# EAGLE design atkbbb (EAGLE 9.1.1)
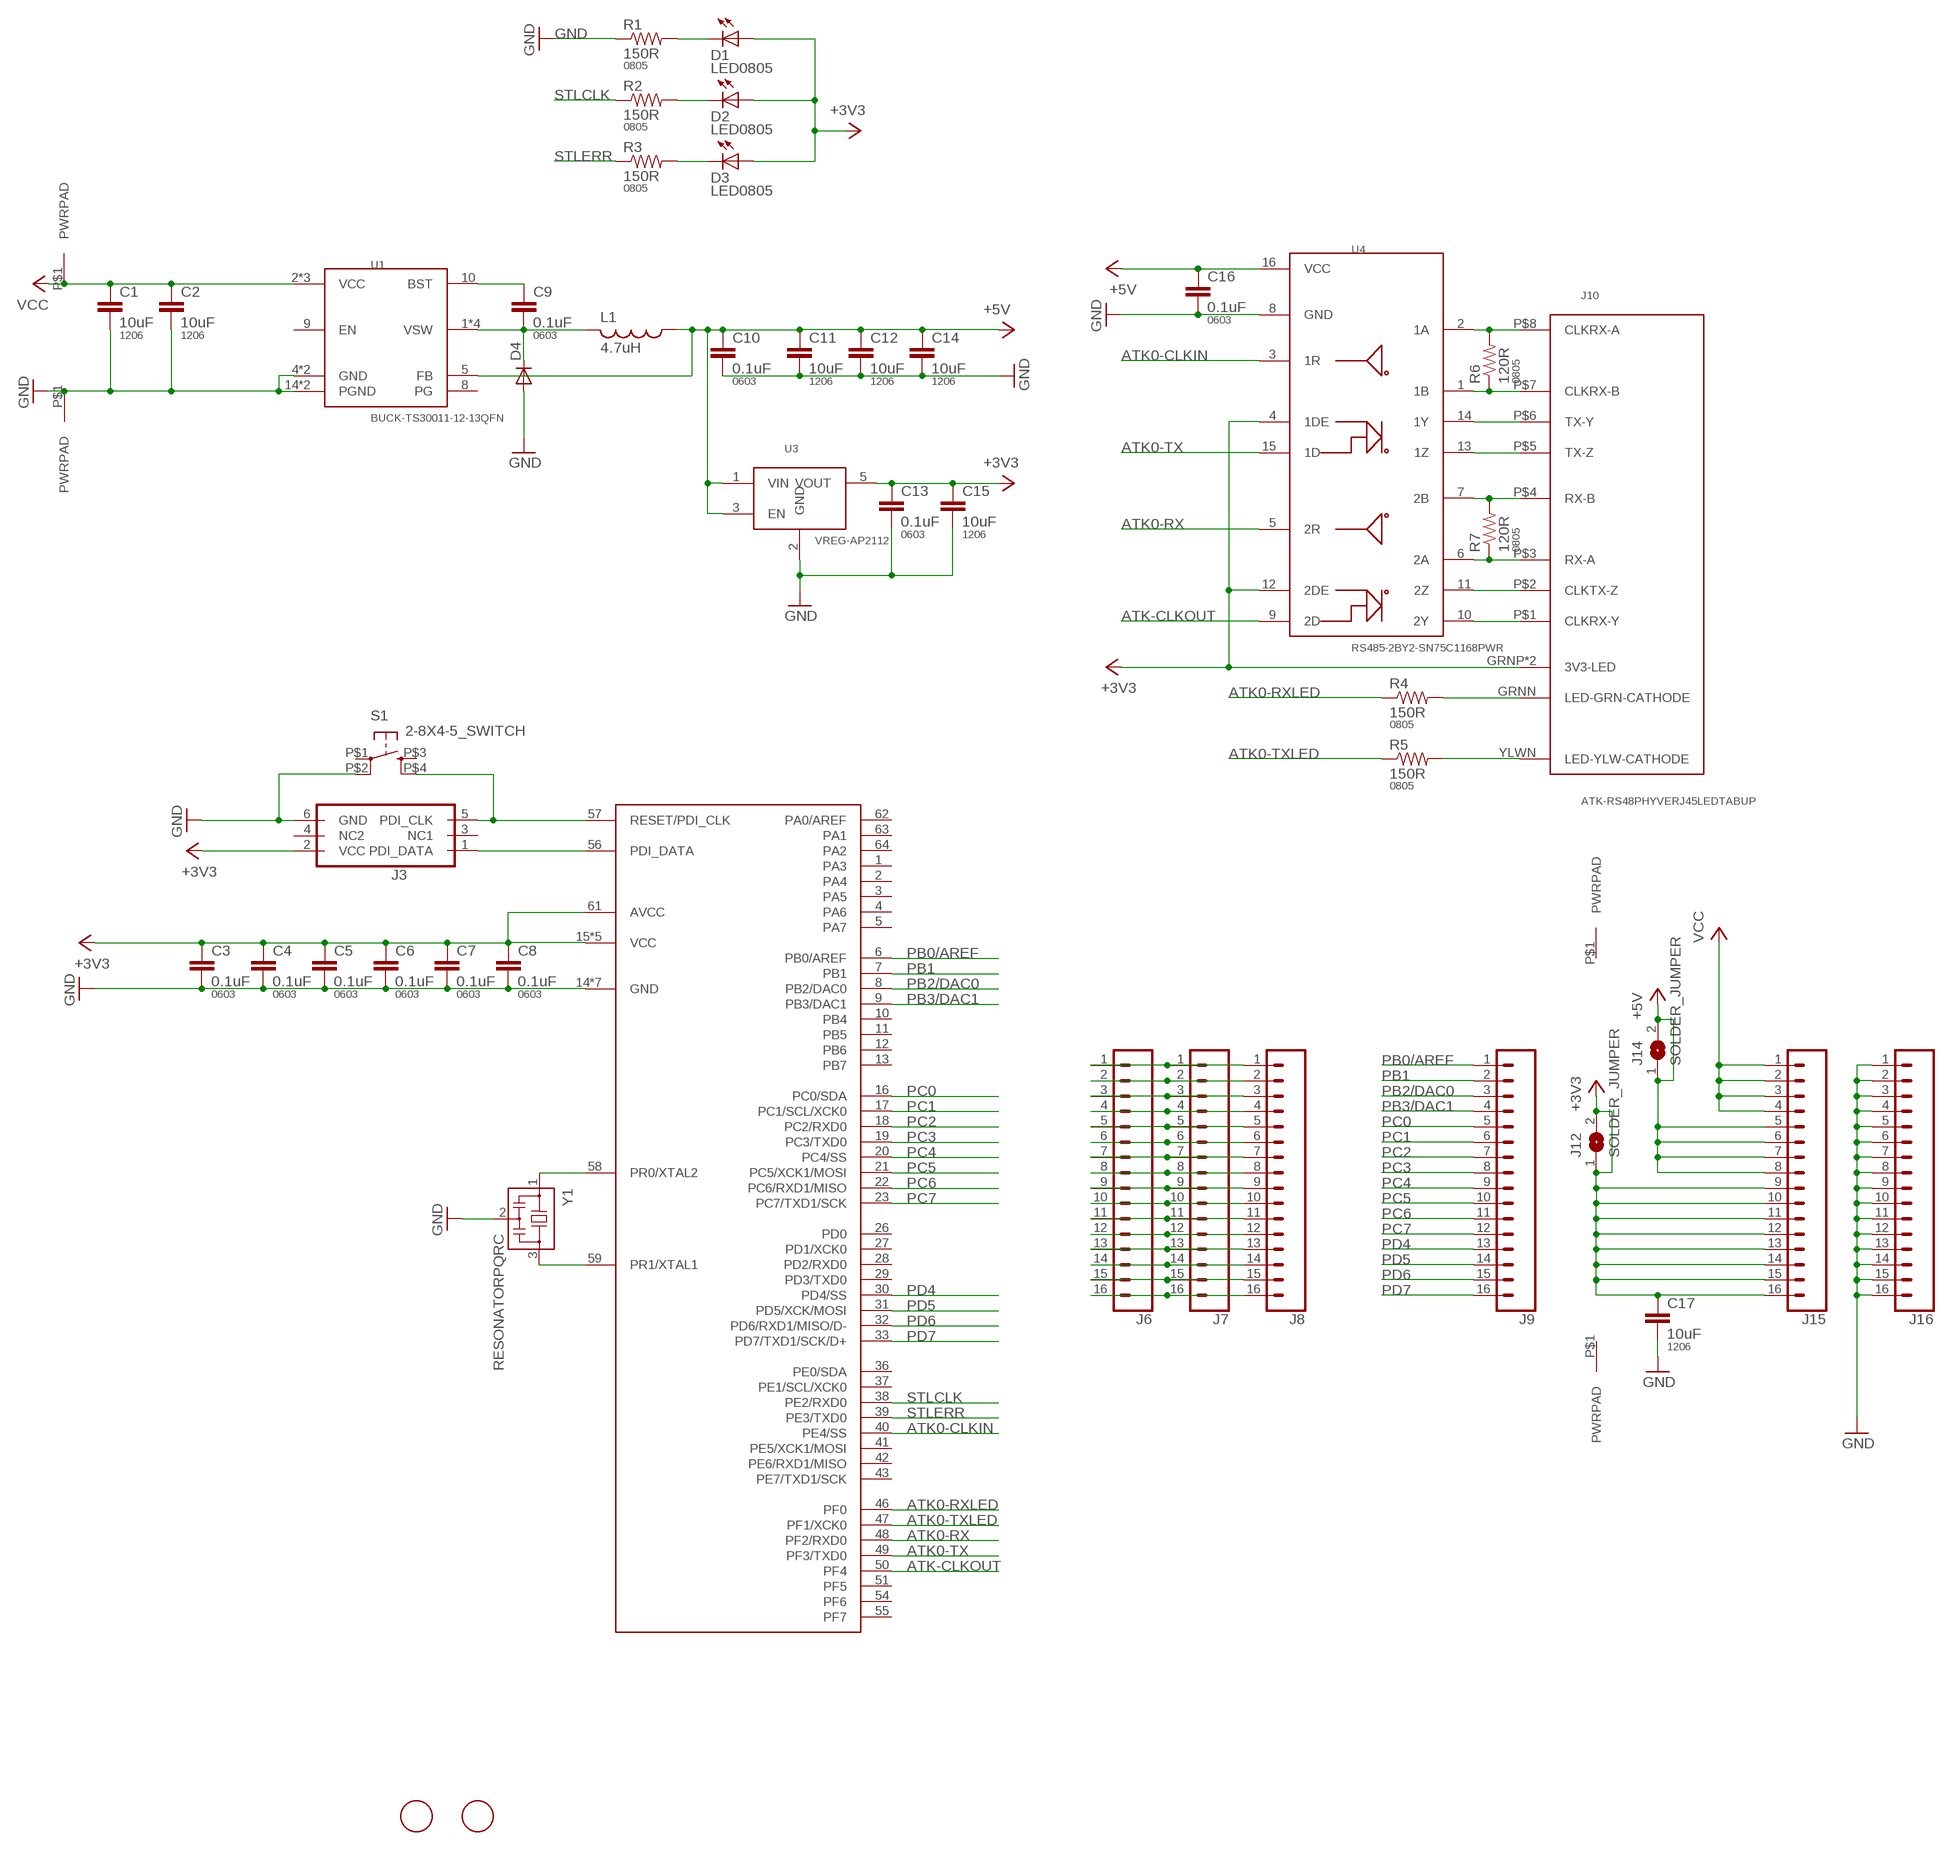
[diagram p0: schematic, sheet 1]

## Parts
C1  10uF  CAP1206  [1206]
C2  10uF  CAP1206  [1206]
C3  0.1uF  CAP0603-CAP  [0603-CAP]
C4  0.1uF  CAP0603-CAP  [0603-CAP]
C5  0.1uF  CAP0603-CAP  [0603-CAP]
C6  0.1uF  CAP0603-CAP  [0603-CAP]
C7  0.1uF  CAP0603-CAP  [0603-CAP]
C8  0.1uF  CAP0603-CAP  [0603-CAP]
C9  0.1uF  CAP0603-CAP  [0603-CAP]
C10  0.1uF  CAP0603-CAP  [0603-CAP]
C11  10uF  CAP1206  [1206]
C12  10uF  CAP1206  [1206]
C13  0.1uF  CAP0603-CAP  [0603-CAP]
C14  10uF  CAP1206  [1206]
C15  10uF  CAP1206  [1206]
C16  0.1uF  CAP0603-CAP  [0603-CAP]
C17  10uF  CAP1206  [1206]
D1  LED0805  [LED0805]
D2  LED0805  [LED0805]
D3  LED0805  [LED0805]
D4  DIODESOD123HE  [SOD-123HE]
J1  PWRPADM3-STANDOFF  [PWRPAD_M3_STANDOFF]
J2  PWRPADM3-STANDOFF  [PWRPAD_M3_STANDOFF]
J3  PDIFEMALE_SMD  [PDI_2X3_SMD]
J4  FIDUCIAL  [FIDUCIAL_1MM]
J5  FIDUCIAL  [FIDUCIAL_1MM]
J6  CONN_161X16_NO_SILK  [1X16_NO_SILK]
J7  CONN_161X16_NO_SILK  [1X16_NO_SILK]
J8  CONN_161X16_NO_SILK  [1X16_NO_SILK]
J9  CONN_161X16_NO_SILK  [1X16_NO_SILK]
J10  ATK-RS48PHYVERJ45LEDTABUP  [RJ45-LED-RJHSE-5381-UPTAB]
J11  PWRPADM3  [PWRPAD_3-25MM]
J12  SOLDER_JUMPER  [SJFAB]
J13  PWRPADM3  [PWRPAD_3-25MM]
J14  SOLDER_JUMPER  [SJFAB]
J15  CONN_161X16_NO_SILK  [1X16_NO_SILK]
J16  CONN_161X16_NO_SILK  [1X16_NO_SILK]
L1  4.7uH  INDUCTOR  [NRS5020T4R7MMGJ]
R1  150R  RESISTOR0805-RES  [0805]
R2  150R  RESISTOR0805-RES  [0805]
R3  150R  RESISTOR0805-RES  [0805]
R4  150R  RESISTOR0805-RES  [0805]
R5  150R  RESISTOR0805-RES  [0805]
R6  120R  RESISTOR0805-RES  [0805]
R7  120R  RESISTOR0805-RES  [0805]
S1  2-8X4-5_SWITCH  [TACT-SWITCH-KMR6]
U1  BUCK-TS30011-12-13QFN  [QFN16-3X3-TI-RTE]
U2  ATXMEGA_A3UQFN  [QFN-64-9X9MM]
U3  VREG-AP2112  [SOT23-5]
U4  RS485-2BY2-SN75C1168PWR  [TSSOP16]
Y1  RESONATORPQRC  [RES_PRQC]

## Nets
+3V3: C3.1 C4.1 C5.1 C6.1 C7.1 C8.1 C13.1 C15.1 C17.1 D1.1(A) D2.1(A) D3.1(A) J3.2(VCC) J10.GRNP(3V3-LED) J10.YLWP(3V3-LED) J12.1 J12.2 J15.9 J15.10 J15.11 J15.12 J15.13 J15.14 J15.15 J15.16 U2.15(VCC) U2.25(VCC) U2.35(VCC) U2.45(VCC) U2.53(VCC) U2.61(AVCC) U3.5(VOUT) U4.4(1DE) U4.12(2DE)
+5V: C10.1 C11.1 C12.1 C14.1 C16.1 J14.1 J14.2 J15.5 J15.6 J15.7 J15.8 L1.1 U1.5(FB) U3.1(VIN) U3.3(EN) U4.16(VCC)
ATK0-CLKIN: U2.40(PE4/SS) U4.3(1R)
ATK0-RX: U2.48(PF2/RXD0) U4.5(2R)
ATK0-RXLED: R4.1 U2.46(PF0)
ATK0-TX: U2.49(PF3/TXD0) U4.15(1D)
ATK0-TXLED: R5.1 U2.47(PF1/XCK0)
ATK-CLKOUT: U2.50(PF4) U4.9(2D)
GND: C1.2 C2.2 C3.2 C4.2 C5.2 C6.2 C7.2 C8.2 C10.2 C11.2 C12.2 C13.2 C14.2 C15.2 C16.2 C17.2 D4.P$2(A) J2.P$1(PWRPAD) J3.6(GND) J16.1 J16.2 J16.3 J16.4 J16.5 J16.6 J16.7 J16.8 J16.9 J16.10 J16.11 J16.12 J16.13 J16.14 J16.15 J16.16 R1.1 S1.P$2(P1) U1.4(GND) U1.14(PGND) U1.15(PGND) U1.TH(GND) U2.14(GND) U2.24(GND) U2.34(GND) U2.44(GND) U2.52(GND) U2.60(GND) U2.P$1(GND) U3.2(GND) U4.8(GND) Y1.2
N$1: U2.58(PR0/XTAL2) Y1.1
N$2: U2.59(PR1/XTAL1) Y1.3
N$3: J3.5(PDI_CLK) S1.P$4(S1) U2.57(RESET/PDI_CLK)
N$4: J3.1(PDI_DATA) U2.56(PDI_DATA)
N$5: C9.1 U1.10(BST)
N$6: C9.2 D4.P$1(C) L1.2 U1.1(VSW) U1.12(VSW) U1.13(VSW) U1.16(VSW)
N$7: J10.GRNN(LED-GRN-CATHODE) R4.2
N$8: J10.P$8(CLKRX-A) R6.2 U4.2(1A)
N$9: D1.2(C) R1.2
N$10: D2.2(C) R2.2
N$11: D3.2(C) R3.2
N$12: J10.P$7(CLKRX-B) R6.1 U4.1(1B)
N$13: J10.P$6(TX-Y) U4.14(1Y)
N$14: J10.P$5(TX-Z) U4.13(1Z)
N$15: J10.P$4(RX-B) R7.2 U4.7(2B)
N$16: J10.P$3(RX-A) R7.1 U4.6(2A)
N$17: J10.P$2(CLKTX-Z) U4.11(2Z)
N$18: J10.P$1(CLKRX-Y) U4.10(2Y)
N$19: J10.YLWN(LED-YLW-CATHODE) R5.2
N$20: J6.1 J7.1 J8.1
N$21: J6.2 J7.2 J8.2
N$22: J6.3 J7.3 J8.3
N$23: J6.4 J7.4 J8.4
N$24: J6.5 J7.5 J8.5
N$25: J6.6 J7.6 J8.6
N$26: J6.7 J7.7 J8.7
N$27: J6.8 J7.8 J8.8
N$28: J6.9 J7.9 J8.9
N$29: J6.10 J7.10 J8.10
N$30: J6.11 J7.11 J8.11
N$31: J6.12 J7.12 J8.12
N$32: J6.13 J7.13 J8.13
N$33: J6.14 J7.14 J8.14
N$34: J6.15 J7.15 J8.15
N$35: J6.16 J7.16 J8.16
PB0/AREF: J9.1 U2.6(PB0/AREF)
PB1: J9.2 U2.7(PB1)
PB2/DAC0: J9.3 U2.8(PB2/DAC0)
PB3/DAC1: J9.4 U2.9(PB3/DAC1)
PC0: J9.5 U2.16(PC0/SDA)
PC1: J9.6 U2.17(PC1/SCL/XCK0)
PC2: J9.7 U2.18(PC2/RXD0)
PC3: J9.8 U2.19(PC3/TXD0)
PC4: J9.9 U2.20(PC4/SS)
PC5: J9.10 U2.21(PC5/XCK1/MOSI)
PC6: J9.11 U2.22(PC6/RXD1/MISO)
PC7: J9.12 U2.23(PC7/TXD1/SCK)
PD4: J9.13 U2.30(PD4/SS)
PD5: J9.14 U2.31(PD5/XCK/MOSI)
PD6: J9.15 U2.32(PD6/RXD1/MISO/D-)
PD7: J9.16 U2.33(PD7/TXD1/SCK/D+)
STLCLK: R2.1 U2.38(PE2/RXD0)
STLERR: R3.1 U2.39(PE3/TXD0)
VCC: C1.1 C2.1 J1.P$1(PWRPAD) J15.1 J15.2 J15.3 J15.4 U1.2(VCC) U1.3(VCC) U1.11(VCC)
Unconnected: J3.3(NC1) J3.4(NC2) J11.P$1(PWRPAD) J13.P$1(PWRPAD) S1.P$1(P) S1.P$3(S) U1.8(PG) U1.9(EN) U2.1(PA3) U2.2(PA4) U2.3(PA5) U2.4(PA6) U2.5(PA7) U2.10(PB4) U2.11(PB5) U2.12(PB6) U2.13(PB7) U2.26(PD0) U2.27(PD1/XCK0) U2.28(PD2/RXD0) U2.29(PD3/TXD0) U2.36(PE0/SDA) U2.37(PE1/SCL/XCK0) U2.41(PE5/XCK1/MOSI) U2.42(PE6/RXD1/MISO) U2.43(PE7/TXD1/SCK) U2.51(PF5) U2.54(PF6) U2.55(PF7) U2.62(PA0/AREF) U2.63(PA1) U2.64(PA2)

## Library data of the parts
C1 C2 C11 C12 C14 C15 C17 = borkedlabs-passives:CAP: Capacitor; PACKAGE: 1206
C3-C10 C13 C16 = borkedlabs-passives:CAP: Capacitor; PACKAGE: 0603
D1-D3 = lights:LED: LED
D4 = passives:DIODE: DIODE
J1 J2 J11 J13 = power:PWRPAD
J3 = microcontrollers:PDI: Multi connection point. Often used as Generic Header-pin footprint for 0.1 inch spaced/style header connections You can populate with any combo of single row headers, but if you'd like an exact match, check these: Header - 2x3 (Male, 0.1") (PRT-12807) Header - 2x3 (Female, 0.1") (PRT-13010) 2x3 Pin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; PROD_ID: CONN-11290
J4 J5 = connector:FIDUCIAL: For use by pick and place machines to calibrate the vision/machine, 1mm
J6-J9 J15 J16 = SparkFun-Connectors:CONN_16: Multi connection point. Often used as Generic Header-pin footprint for 0.1 inch spaced/style header connections On any of the 0.1 inch spaced packages, you can populate with these: Break Away Headers - Straight (PRT-00116) Break Away Male Headers - Right Angle (PRT-00553) Female Headers (PRT-00115)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
J10 = connector:ATK-RS48PHYVE
J12 J14 = connector:SOLDER_JUMPER
L1 = power:INDUCTOR
R1-R7 = borkedlabs-passives:RESISTOR: Resistor; PACKAGE: 0805
S1 = passives:2-8X4-5_SWITCH
U1 = power:BUCK-TS30011-12-13
U2 = microcontrollers:ATXMEGA_A3U
U3 = power:VREG-AP2112
U4 = comm:RS485-2BY2-SN75C1168PWR
Y1 = passives:RESONATOR

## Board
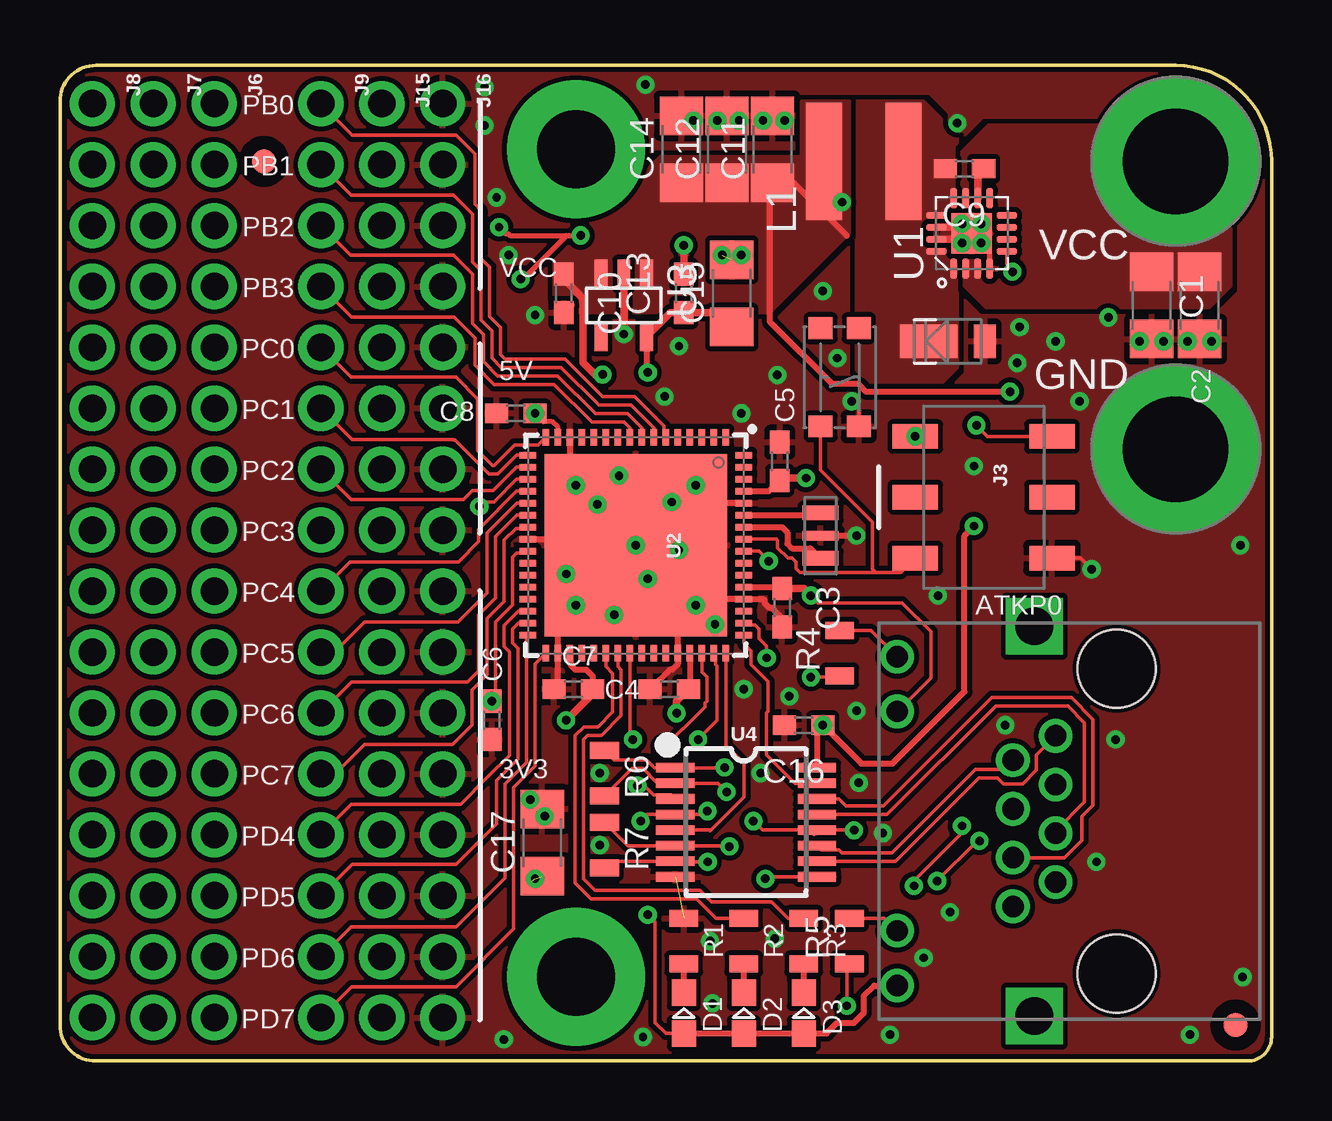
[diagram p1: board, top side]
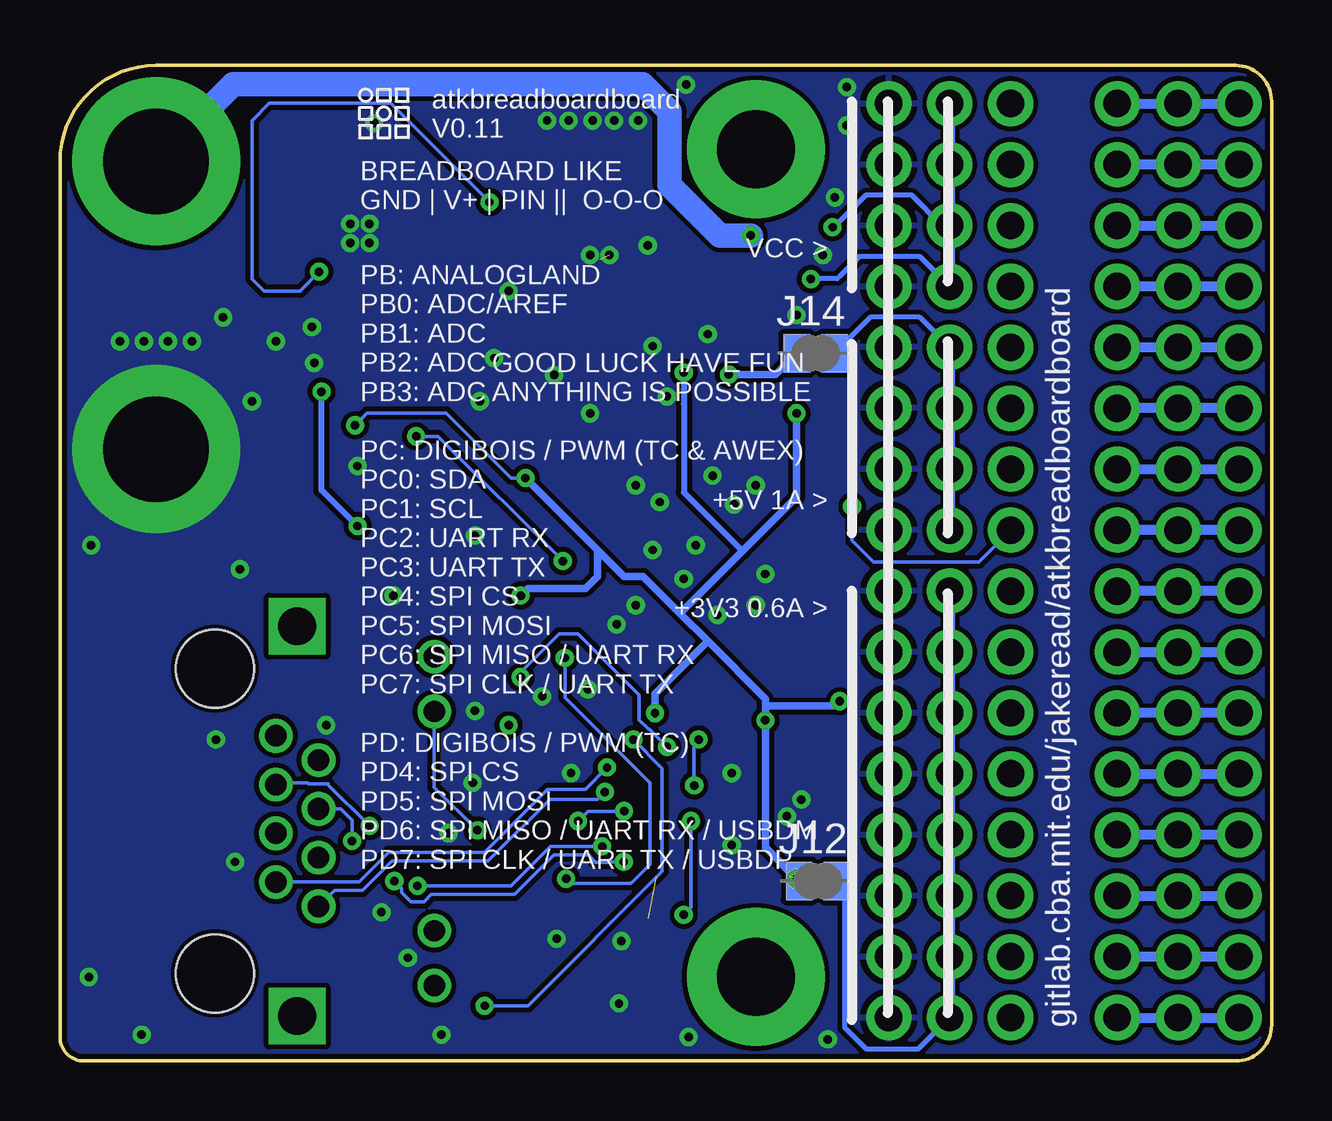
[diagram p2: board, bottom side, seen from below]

Size 50.5 x 41.5 mm. Coordinates in mm from the lower left corner, seen from the top.
Outline: 46.5,41.5 1.5,41.5 arc90 0,40 0,1.5 arc90 1.5,0 49.5,0 arc90 50.5,1 50.5,37.5 arc90 46.5,41.5
Copper layers (1*16): Top 0.035mm / dielectric 1.5mm / Bottom 0.035mm
Design rules "default *": minimum track width 6mil, minimum drill 0.35mm, track to track 8mil, track to pad 8mil, pad to pad 8mil, via to via 8mil, smd to smd 8mil, copper to edge 8mil, drill to drill 8mil, minimum pad ring 10mil, minimum via ring 8mil, stop-mask expansion 4mil, vias tented up to drill 25mil, thermal gap 10mil

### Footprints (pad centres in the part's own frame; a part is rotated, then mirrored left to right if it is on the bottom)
1206 = smd 1.6 x 1.8: 1 -1.4,0; 2 1.4,0
0603-CAP = smd 0.96 x 0.8: 1 -0.8,0; 2 0.8,0
LED0805 = smd 1.1 x 1: 1 -0.85,0; 2 0.85,0
SOD-123HE = smd 2.4 x 1.4: P$1 0.8,0 | smd 0.9 x 1.4: P$2 -1.55,0
PWRPAD_M3_STANDOFF = drill 4.4 pad 7: P$1 0,0
PDI_2X3_SMD = smd 1.02 x 1.9: 1 -2.54,-2.85; 2 -2.54,2.85; 3 0,-2.85; 4 0,2.85; 5 2.54,-2.85; 6 2.54,2.85
FIDUCIAL_1MM = smd 1 x 1: 1 0,0
1X16_NO_SILK = drill 1.143 pad 1.88: 1 0,0; 2 2.54,0; 3 5.08,0; 4 7.62,0; 5 10.16,0; 6 12.7,0; 7 15.24,0; 8 17.78,0; 9 20.32,0; 10 22.86,0; 11 25.4,0; 12 27.94,0; 13 30.48,0; 14 33.02,0; 15 35.56,0; 16 38.1,0
RJ45-LED-RJHSE-5381-UPTAB = drill 0.889: GRNN 6.858,6.604; GRNP 4.572,6.604; YLWN -4.572,6.604; YLWP -6.858,6.604 | drill 0.9: P$1 3.556,0; P$2 2.54,1.778; P$3 1.524,0; P$4 0.508,1.778; P$5 -0.508,0; P$6 -1.524,1.778; P$7 -2.54,0; P$8 -3.556,1.778 | drill 1.575 square: SHDL1 -8.128,0.889; SHDL2 8.128,0.889 | hole 3.251: -6.35,-2.54; 6.35,-2.54
PWRPAD_3-25MM = drill 3.25 pad 5.75: P$1 0,0
SJFAB = smd 1.118 x 1.6: 1 -0.787,0; 2 0.787,0
NRS5020T4R7MMGJ = smd 4.9 x 1.5: 1 0,1.65; 2 0,-1.65
0805 = smd 0.7 x 1.2: 1 -0.95,0; 2 0.95,0
TACT-SWITCH-KMR6 = smd 0.9 x 1: P$1 -2.05,0.8; P$2 2.05,0.8; P$3 -2.05,-0.8; P$4 2.05,-0.8
QFN16-3X3-TI-RTE = smd 0.85 x 0.3: 1 -1.475,0.75; 2 -1.475,0.25; 3 -1.475,-0.25; 4 -1.475,-0.75; 9 1.475,-0.75; 10 1.475,-0.25; 11 1.475,0.25; 12 1.475,0.75 | smd 0.3 x 0.85: 5 -0.75,-1.475; 6 -0.25,-1.475; 7 0.25,-1.475; 8 0.75,-1.475; 13 0.75,1.475; 14 0.25,1.475; 15 -0.25,1.475; 16 -0.75,1.475 | smd 1.7 x 1.7: TH 0,0
QFN-64-9X9MM = smd 0.7 x 0.275: 1 -4.5,3.75; 2 -4.5,3.25; 3 -4.5,2.75; 4 -4.5,2.25; 5 -4.5,1.75; 6 -4.5,1.25; 7 -4.5,0.75; 8 -4.5,0.25; 9 -4.5,-0.25; 10 -4.5,-0.75; 11 -4.5,-1.25; 12 -4.5,-1.75; 13 -4.5,-2.25; 14 -4.5,-2.75; 15 -4.5,-3.25; 16 -4.5,-3.75; 33 4.5,-3.75; 34 4.5,-3.25; 35 4.5,-2.75; 36 4.5,-2.25; 37 4.5,-1.75; 38 4.5,-1.25; 39 4.5,-0.75; 40 4.5,-0.25; 41 4.5,0.25; 42 4.5,0.75; 43 4.5,1.25; 44 4.5,1.75; 45 4.5,2.25; 46 4.5,2.75; 47 4.5,3.25; 48 4.5,3.75 | smd 0.275 x 0.7: 17 -3.75,-4.5; 18 -3.25,-4.5; 19 -2.75,-4.5; 20 -2.25,-4.5; 21 -1.75,-4.5; 22 -1.25,-4.5; 23 -0.75,-4.5; 24 -0.25,-4.5; 25 0.25,-4.5; 26 0.75,-4.5; 27 1.25,-4.5; 28 1.75,-4.5; 29 2.25,-4.5; 30 2.75,-4.5; 31 3.25,-4.5; 32 3.75,-4.5; 49 3.75,4.5; 50 3.25,4.5; 51 2.75,4.5; 52 2.25,4.5; 53 1.75,4.5; 54 1.25,4.5; 55 0.75,4.5; 56 0.25,4.5; 57 -0.25,4.5; 58 -0.75,4.5; 59 -1.25,4.5; 60 -1.75,4.5; 61 -2.25,4.5; 62 -2.75,4.5; 63 -3.25,4.5; 64 -3.75,4.5 | smd 7.6 x 7.6: P$1 0,0
SOT23-5 = smd 0.533 x 1.194: 1 -0.95,-1.306; 2 0,-1.306; 3 0.95,-1.306; 4 0.95,1.306; 5 -0.95,1.306
TSSOP16 = smd 0.4 x 1.6: 1 -2.225,-2.85; 2 -1.575,-2.85; 3 -0.925,-2.85; 4 -0.275,-2.85; 5 0.375,-2.85; 6 1.025,-2.85; 7 1.675,-2.85; 8 2.325,-2.85; 9 2.325,3.05; 10 1.675,3.05; 11 1.025,3.05; 12 0.375,3.05; 13 -0.275,3.05; 14 -0.925,3.05; 15 -1.575,3.05; 16 -2.225,3.05
RES_PRQC = smd 0.6 x 1.5: 1 -0.95,0; 3 0.95,0 | smd 0.4 x 1.5: 2 0,0

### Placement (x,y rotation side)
C1  45.5,31.5 270 top
C2  47.5,31.5 270 top
C3  30.1,18.9 270 top
C4  25.4,15.5 180 top
C5  30,25 90 top
C6  18,14.2 270 top
C7  21.4,15.5 180 top
C8  19,27 180 top
C9  37.7,37.2 180 top
C10  21,32 270 top
C11  29.7,38 90 top
C12  27.8,38 90 top
C13  26,32 90 top
C14  25.9,38 90 top
C15  28,32 90 top
C16  31,14 180 top
C17  20.1,9.1 90 top
D1  26,2 90 top
D2  28.5,2 90 top
D3  31,2 90 top
D4  37,30 180 top
J1  46.5,37.5 0 top
J2  46.5,25.5 0 top
J3  38.5,23.5 270 top
J4  8.5,37.5 0 top
J5  49,1.5 0 top
J6  6.43,39.91 270 top
J7  3.89,39.91 270 top
J8  1.35,39.91 270 top
J9  10.88,39.91 270 top
J10  41.5,10 90 top
J11  21.5,3.5 0 top
J12  18.9,7.5 0 bottom
J13  21.5,38 180 top
J14  19,29.5 0 bottom
J15  13.41,39.91 270 top
J16  15.96,39.91 270 top
L1  33.5,37.5 90 top
R1  26,5 270 top
R2  28.5,5 270 top
R3  31,5 270 top
R4  32.5,17 90 top
R5  32.9,5 90 top
R6  22.7,12 270 top
R7  22.7,9 270 top
S1  32.5,28.5 270 top
U1  38,34.5 90 top
U2  24,21.5 270 top
U3  23.5,31.5 180 top
U4  28.5,10 270 top
U$6  CBA-LOGO  [CBA-SILK-LOGO]  37,39.5 0 bottom
Y1  31.7,21.9 90 top

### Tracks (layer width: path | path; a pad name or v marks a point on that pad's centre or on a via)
+3V3  (via drill 0.35)  (2 unrouted)
  Top 0.152: v24.2,10 24.48,10.28 U4.4 26.84,10.28 v26.98,10.41 | v24.5,6.1 24.8,5.8 24.8,1.6 25.25,1.15 D1.1 | U4.12 31.52,9.6 | U2.25 19.42,21.17 19.03,21.17 18.87,21 18.87,19.01 18.16,18.3 18.16,15.16 C6.1 | v28.9,10 29.27,9.62 U4.12 | U4.12 v33.09,9.62 v33.1,9.62 | v31.3,19.4 31.6,19.1 35.1,19.1 36.3,17.9 36.3,15.98 J10.GRNP | v38.2,26.5 38.66,26.04 J3.2
  Top 0.203: C8.1 20.14,26.66 20.51,26.66 20.75,26.42 U2.15
  Top 0.254: U2.61 29.55,23.75 C5.1 | C7.1 22.2,16.05 21.93,16.32 21.48,16.32 21.28,16.51 21.28,16.97 U2.35 | U2.45 26.25,15.55 C4.1 | U2.53 30.05,19.75 C3.1 | U4.12 31.43,9.51 | D1.1 D2.1 D3.1 31.95,1.15 32.09,1.29 | 32.09,1.29 | J10.YLWP 33.94,3.14 33.51,2.71 33.51,2.01 33.09,1.59 32.39,1.59 32.09,1.29 | U3.5 24.45,28.75 v24.5,28.7
  Top 0.305: C15.1 27.4,31.2 C13.1 25.46,31.2 U3.5 | C5.1 30.1,24.3 v31.1,24.3 | C3.1 31,19.7 v31.3,19.4 | v21.1,14.2 22.2,15.3 C7.1 | v25.7,14.5 25.7,15 C4.1
  Bottom 0.152: v24.2,10 24.2,6.4 v24.5,6.1 | v26.98,10.41 28.48,10.41 v28.9,10 | v33.1,9.62 34.9,11.41 J10.GRNP | v31.1,24.3 31.7,24.3 34.4,27 37.7,27 v38.2,26.5
  Bottom 0.203: 13.48,8.13 13.41,8.2 | J12.2 17.8,7.19 17.8,1.4 16.9,0.5 14.72,0.5 J15.16
  Bottom 0.254: 22.05,21.25 24.5,23.7 24.5,27.4 24.49,27.41 24.49,27.99 24.5,28 v24.5,28.7
  Bottom 0.305: v31.3,19.4 31,19.7 28.6,19.7 28.1,20.2 28.1,21.3 | v31.1,24.3 28.1,21.3 | 28.1,21.3 27,20.2 26.2,20.2 24.65,18.65 | 24.65,18.65 23.5,17.5 | 23.5,17.5 21.1,15.1 21.1,14.8 | 21.1,14.8 v21.1,14.2 21.1,8.9 v19.8,7.6 | 23.5,17.5 25.7,15.3 v25.7,14.5 | 21.1,14.8 18.2,14.8 C6.1 | C8.1 19.8,23.5 22.05,21.25 24.65,18.65
  Bottom 0.406: J15.9 J15.10 J15.11 J15.12 J15.13 13.41,8.2 J15.14 J15.15 J15.16
  Bottom 0.813: J12.1 J12.2
  other vias: 18,15 19.8,27
+5V  (via drill 0.35)
  Top 0.152: U1.5 39.48,33.23 39.7,33 v39.7,32.9
  Top 0.254: 32.8,34.4 30.6,36.6 C11.1 29.6,36.5 29.6,30.8 32.19,28.21 33.29,28.21 33.6,27.9 v39.6,27.9 | U4.16 31.55,13.75 C16.1 33.4,12.4 34.7,12.4 37.7,15.4 37.7,21.9 v38.1,22.3
  Top 0.305: C10.1 21,32.58 21.81,31.77 21.81,31.29 21.8,31.28 21.8,29.12 22.36,28.56 22.56,28.56 v22.62,28.62
  Bottom 0.152: v32.6,35.8 36.73,39.92 41.77,39.92 42.5,39.2 42.5,32.6 42,32.1 40.5,32.1 v39.7,32.9
  Bottom 0.203: J15.5 14.66,31 16.71,31 J14.2
  Bottom 0.254: v38.1,22.3 39.6,23.8 v39.6,27.9
  Bottom 0.305: v22.62,28.62 20.67,28.62 J14.1
  Bottom 0.406: J15.5 J15.6 13.41,25.9 J15.7 J15.8
  Bottom 0.813: J14.1 J14.2
  other vias: 31.8,14
  pour Top (no thermals): 32.9,40 30.9,40 30.9,37.7 25,37.7 23,35.7 21.6,35.7 20.6,34.7 20.6,31.2 29.6,31.2 32.9,34.5
ATK0-CLKIN  (via drill 0.35)
  Top 0.152: U4.3 25.48,11.1 24.73,11.1 24.34,11.48 v24.07,11.48 | U2.40 23.75,13.53 v23.88,13.4
  Bottom 0.152: v24.07,11.48 24.07,13.22 v23.88,13.4
ATK0-RX
  Top 0.152: U2.48 27.75,13.15 28.5,12.4 28.5,11 27.1,9.6 27.07,9.62 U4.5
ATK0-RXLED  (via drill 0.35)
  Top 0.152: 32.45,16.1 R4.1 32.45,16 v31.3,16 | v25.2,13.1 25.94,13.84 25.97,13.84 26.89,14.76 26.89,14.92 26.96,14.98 26.96,16.02 26.75,16.23 U2.46
  Bottom 0.152: v31.3,16 31.3,16.2 29.7,17.8 28.9,17.8 26.36,15.26 26.36,14.23 25.97,13.84 25.94,13.84 v25.2,13.1
ATK0-TX
  Top 0.152: U2.49 28.5,17.4 28.8,17.1 28.8,16.53 29.5,15.83 29.5,14.57 29.44,14.52 29.44,12.76 29.55,12.65 30.62,11.57 U4.15
ATK0-TXLED  (via drill 0.35)
  Top 0.152: v32.8,2.3 32.8,3.95 R5.1 | U2.47 27.33,16.92 27.33,16.53 27.39,16.47 27.39,14.19 v26.6,13.4
  Bottom 0.152: v32.8,2.3 31,2.3 25.4,7.9 25.4,12.2 v26.6,13.4
ATK-CLKOUT  (via drill 0.35)
  Top 0.152: 32.3,7.67 U4.9 29.48,7.67 v29.4,7.6 | v29.46,16.8 29.46,17.29 29.13,17.62 29.13,18 28.97,18.17 28.58,18.17 U2.50
  Bottom 0.152: v29.4,7.6 29.2,7.4 26.7,7.4 25.9,8.2 25.9,11.6 29.46,15.16 v29.46,16.8
GND  (via drill 0.35)  (2 unrouted)
  Top 0.152: S1.P$2 33.3,27.2 v33,27.5 | J3.6 42.54,20.96 v43,20.5
  Top 0.203: U1.4 38.75,33.75 v38.4,34.1
  Top 0.254: U2.60 27.25,23.25 v26.5,24 | v21.5,19 20.75,18.25 U2.34 20.75,15.65 C7.2 | U2.24 23.75,21.75 U2.P$1 | U2.14 21.25,24.25 v21.5,24 | C4.2 25.42,16.32 25.52,16.32 25.75,16.55 U2.44 25.75,18.25 v26.5,19 26.75,19.25 U2.52 29.32,19.25 29.37,19.2 29.37,19.08 29.56,18.89 29.68,18.89 30.1,18.47 C3.2 | Y1.2 v33.2,21.9
  Top 0.305: U1.14 37.75,34.75 U1.TH | U1.15 37.75,34.25 U1.TH | v38.4,34.1 U1.TH | C10.2 21.3,31.5 | C13.2 v26,34 | U3.2 v23.5,30.3
  other vias: 37.6,34.9 37.6,34.1 38.4,34.9 41.5,30 27.6,33.6 28.4,33.6 26.4,39.2 27.4,39.2 28.3,39.2 29.3,39.2 30.2,39.2 24,21.5 45,30 46,30 47,30 48,30 27.2,2.4 24.3,1 37.4,39.1 24.4,40.7 19.6,10.9 20.2,10.2 25.2,27.7 28.4,27 19.8,31.1 18.7,33.6 18.2,36 17.7,40.6 17.7,39 25.8,29.8 31.8,32.1 34.6,1.1 27.1,5 29.8,5.1 23.1,18.6 24.5,20.1 23.3,24.4 27.3,18.2 34.3,9.5 39.4,14 29.2,12 28.5,15.5 33.2,14.6 36.6,19.4 30.4,15.2 33.3,11.6 37.1,6.2 43.2,8.3 44,13.4 36,4.3 47.1,1.1 49.3,3.5 49.2,21.5 38.1,24.8 29.9,28.6 32.4,29.3 40,30.6 39.9,29.1 43.7,31 42.5,27.5 21.1,20.3 25.8,21.3 22.4,23.2 25.5,23.3 22.5,12 22.5,9 18.5,0.9
  pour Top (rank 6): -1,52 -1,-2 52,-2 52,53.5 -0.5,53.5 -0.5,52.5
  pour Bottom (rank 6): -1,54 -1,-2.5 52.5,-2.5 52.5,54
N$1
  Top 0.254: U2.58 30.1,22.25 30.32,22.03 30.32,21.56 30.51,21.37 31.28,21.37 Y1.1
N$2
  Top 0.254: U2.59 31.6,22.75 Y1.3
N$3
  Top 0.152: U2.57 29.86,21.75 29.91,21.7 29.91,21.39 30.34,20.96 30.51,20.96 30.67,20.8 30.67,20.53 30.83,20.37 34,20.37 | J3.5 35.06,20.37 34,20.37 | S1.P$4 31.7,24.63 33.86,22.47 33.86,20.51 34,20.37
N$4  (via drill 0.35)
  Top 0.152: U2.56 29.13,21.25 v29.54,20.84
  Bottom 0.152: J3.1 34.74,26.04 v29.54,20.84
  other vias: 35.65,26.04
N$5
  Top 0.305: U1.10 38.25,36.95 C9.1
N$6
  pour Top (rank 3, no thermals): 33.2,40 33.2,28.8 34.3,27.7 36.2,27.7 37.4,28.9 37.4,38.6 36,40
N$7
  Top 0.152: R4.2 33.8,17.95 J10.GRNN
N$8  (via drill 0.35)
  Top 0.152: R6.2 23.85,12.2 24.3,12.2 24.57,11.93 24.57,11.91 24.91,11.57 U4.2 27.43,11.57 v27.79,11.21
  Bottom 0.152: J10.P$8 39.06,7.1 37.89,7.1 36.65,8.34 32.65,8.34 30.08,10.91 28.09,10.91 v27.79,11.21
N$9
  Top 0.254: D1.2 R1.2
N$10
  Top 0.254: D2.2 R2.2
N$11
  Top 0.254: D3.2 R3.2
N$12  (via drill 0.35)
  Top 0.152: R6.1 23.09,12.56 24.45,12.56 24.78,12.22 U4.1 v27.69,12.22 v27.7,12.23
  Bottom 0.152: J10.P$7 38.04,7.46 36.8,8.7 32.8,8.7 30.17,11.33 28.6,11.33 v27.7,12.23
N$13
  Top 0.152: U4.14 32.48,10.93 32.77,10.63 34.33,10.63 38.85,15.16 42.15,15.16 43.06,14.25 43.06,10.65 42.6,10.2 42.6,9.2 41.88,8.48 J10.P$6
N$14
  Top 0.152: U4.13 34.48,10.28 39,14.8 42,14.8 42.7,14.1 42.7,10.8 41.5,9.6 J10.P$5
N$15  (via drill 0.35)
  Top 0.152: v27,8.3 25.68,8.3 U4.7 22.98,8.32 R7.2 | v36.56,7.5 38.23,9.17 v38.33,9.17
  Bottom 0.152: v27,8.3 27.61,8.3 27.63,8.29 28.17,8.29 28.47,8.59 29.91,8.59 31.55,6.94 35.03,6.94 35.33,6.64 35.87,6.64 36.26,7.03 36.26,7.2 v36.56,7.5 | v38.33,9.17 38.33,10.03 38.81,10.51 J10.P$4
N$16  (via drill 0.35)
  Top 0.152: v27.9,8.94 27.87,8.97 U4.6 23.68,8.97 R7.1 | v35.6,7.3 35.6,7.5 37.6,9.5 v37.6,9.8
  Bottom 0.152: J10.P$3 41.42,11.6 40.17,11.6 40.13,11.56 39.5,11.56 | 39.31,11.56 39.5,11.56 | v27.9,8.94 30.06,8.94 31.7,7.3 v35.6,7.3 | v37.6,9.8 39.36,11.56 39.5,11.56
N$17
  Top 0.152: U4.11 31.72,8.8 32.47,8.8 32.59,8.68 34.68,8.68 38.15,12.16 39.34,12.16 J10.P$2
N$18
  Top 0.152: J10.P$1 40.7,12.76 40.7,12.13 40.13,11.56 39.31,11.56 39.07,11.8 38.3,11.8 34.83,8.32 U4.10
N$19
  Top 0.152: R5.2 34.37,5.95 J10.YLWN
N$20
  Bottom 0.406: J6.1 J7.1 J8.1
N$21
  Bottom 0.406: J8.2 J7.2 J6.2
N$22
  Bottom 0.406: J6.3 J7.3 J8.3
N$23
  Bottom 0.406: J8.4 J7.4 J6.4
N$24
  Bottom 0.406: J6.5 J7.5 J8.5
N$25
  Bottom 0.406: J8.6 J7.6 J6.6
N$26
  Bottom 0.406: J6.7 J7.7 J8.7
N$27
  Bottom 0.406: J8.8 J7.8 J6.8
N$28
  Bottom 0.406: J8.9 J7.9 J6.9
N$29
  Bottom 0.406: J6.10 J7.10 J8.10
N$30
  Bottom 0.406: J8.11 J7.11 J6.11
N$31
  Bottom 0.406: J6.12 J7.12 J8.12
N$32
  Bottom 0.406: J8.13 J7.13 J6.13
N$33
  Bottom 0.406: J6.14 J7.14 J8.14
N$34
  Bottom 0.406: J8.15 J7.15 J6.15
N$35
  Bottom 0.406: J6.16 J7.16 J8.16
PB0/AREF
  Top 0.152: U2.6 25.17,26.08 25.17,26.47 23.95,27.7 23.2,27.7 22.61,27.7 21.04,29.27 18.54,29.27 18.37,29.44 18.37,30.57 17.91,31.03 17.91,33.09 17.56,33.45 17.56,35.46 17.3,35.71 17.3,37.8 16.5,38.6 12.19,38.6 J9.1
PB1
  Top 0.152: J9.2 12.14,36.1 16.41,36.1 17.2,35.31 17.2,33.3 17.56,32.95 17.56,30.88 18.01,30.42 18.01,29.3 18.39,28.91 20.89,28.91 22.46,27.34 23.8,27.34 24.75,26.39 U2.7
PB2/DAC0
  Top 0.152: J9.3 12.11,33.6 16.4,33.6 17.2,32.8 17.2,30.73 17.66,30.28 17.66,29.15 18.25,28.56 20.75,28.56 22.32,26.98 23.65,26.98 24.25,26.39 U2.8
PB3/DAC1
  Top 0.152: J9.4 12.16,31 16.43,31 17.3,30.13 17.3,29 18.1,28.2 20.6,28.2 22.17,26.63 23.5,26.63 23.75,26.38 U2.9
PC0
  Top 0.152: J9.5 12.12,28.5 16.5,28.5 17.4,27.6 17.4,25.45 18.04,24.81 18.09,24.81 18.95,25.67 19.92,25.67 U2.16
PC1
  Top 0.152: J9.6 12.19,25.9 16.4,25.9 16.41,25.89 16.46,25.89 17.89,24.46 18.24,24.46 19.03,25.25 U2.17
PC2
  Top 0.152: J9.7 12.14,23.4 16.83,23.4 17.21,23.78 18.06,23.78 19.04,24.75 U2.18
PC3  (via drill 0.35)
  Top 0.152: v17.48,23.12 17.66,23.3 18.09,23.3 19.04,24.25 U2.19
  Bottom 0.152: J9.8 12.21,20.8 12.9,20.8 12.91,20.81 16.46,20.81 16.47,20.8 16.6,20.8 17.5,21.7 17.48,21.72 v17.48,23.12
PC4
  Top 0.152: J9.9 12.09,20.81 16.61,20.81 17.45,21.65 17.45,22.16 19.04,23.75 U2.20
PC5
  Top 0.152: J9.10 11.45,17.05 12.7,18.3 16.6,18.3 17.8,19.5 17.8,22.01 19.04,23.25 U2.21
PC6
  Top 0.152: J9.11 12.16,15.8 17,15.8 17.45,16.25 17.45,18.59 18.16,19.3 18.16,21.86 19.05,22.75 U2.22
PC7
  Top 0.152: J9.12 11.47,11.97 12.7,13.2 16.37,13.2 17.17,14.01 17.17,15.47 17.8,16.1 17.8,18.45 18.52,19.16 18.52,21.71 19,22.2 19.45,22.2 U2.23
PD4
  Top 0.152: J9.13 12.14,10.7 16.7,10.7 17.83,11.83 17.83,11.84 18.73,12.74 18.73,17.05 18.52,17.27 18.52,18.15 19.11,18.75 U2.30
PD5
  Top 0.152: J9.14 12.19,8.2 16.5,8.2 18.19,9.89 18.19,11.7 19.09,12.6 19.09,17.2 18.87,17.42 18.87,18 19.12,18.25 U2.31
PD6
  Top 0.152: J9.15 12.12,5.6 16.5,5.6 18.54,7.64 18.54,11.55 19.44,12.45 19.44,17.69 U2.32
PD7
  Top 0.152: J9.16 12.16,3.1 16.5,3.1 18.9,5.5 18.9,11.4 19.8,12.3 19.8,16.55 U2.33
STLCLK
  Top 0.152: R2.1 27.34,5.95 26.54,6.76 22.14,6.76 21.46,7.43 21.46,13.56 21.84,13.94 22.43,13.94 23.04,14.55 23.04,16.15 22.75,16.44 U2.38
STLERR
  Top 0.152: R3.1 30.35,5.95 29.66,6.64 27.15,6.64 26.68,7.11 22.29,7.11 21.82,7.58 21.82,13.42 21.98,13.58 22.57,13.58 23.39,14.4 23.39,16.3 23.25,16.44 U2.39
VCC  (via drill 0.35)
  Top 0.203: v19.2,32.6 19.3,32.6 21.11,34.41 21.2,34.41 | 21.2,34.41 v21.7,34.41 | v18.3,34.76 18.58,34.48 18.68,34.48 18.75,34.41 21.2,34.41
  Bottom 0.203: J15.4 14.66,33.53 17.18,33.53 18.01,32.71 18.11,32.61 v19.19,32.61 v19.2,32.6 | J15.3 13.73,34.83 15,36.1 16.9,36.1 18.24,34.76 v18.3,34.76
  Bottom 0.406: J15.1 J15.2 J15.3 J15.4
  Bottom 1.016: v21.7,34.41 22.98,34.41 25.09,36.52 25.09,37.8 25.09,39.59 26.21,40.71 43.29,40.71 J1.P$1
  pour Top (rank 2, no thermals): 37.6,35.5 37.6,37.9 38.7,39 44.5,39 48.8,34.7 48.8,32.3 47.9,31.4 38.6,31.4 37.7,32.3 37.7,35.4

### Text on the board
tPlace: PB0 | PB1 | PB2 | VCC | VCC | PB3 | PC0 | 5V | GND | PC1 | PC2 | PC3 | PC4 | ATKP0 | PC5 | PC6 | 3V3 | PC7 | PD4 | PD5 | PD6 | PD7
bPlace: atkbreadboardboard / V0.11 | BREADBOARD LIKE / GND | V+ | PIN || O-O-O | VCC > | GOOD LUCK HAVE FUN / ANYTHING IS POSSIBLE | +5V 1A > | +3V3 0.6A > | PB: ANALOGLAND / PB0: ADC/AREF / PB1: ADC / PB2: ADC / PB3: ADC / / PC: DIGIBOIS / PWM (TC & AWEX) / PC0: SDA / PC1: SCL / PC2: UART RX / PC3: UART TX / PC4: SPI CS / PC5: SPI MOSI / PC6: SPI MISO / UART RX / PC7: SPI CLK / UART TX / / PD: DIGIBOIS / PWM (TC) / PD4: SPI CS / PD5: SPI MOSI / PD6: SPI MISO / UART RX / USBDM / PD7: SPI CLK / UART TX / USBDP | gitlab.cba.mit.edu/jakeread/atkbreadboardboard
